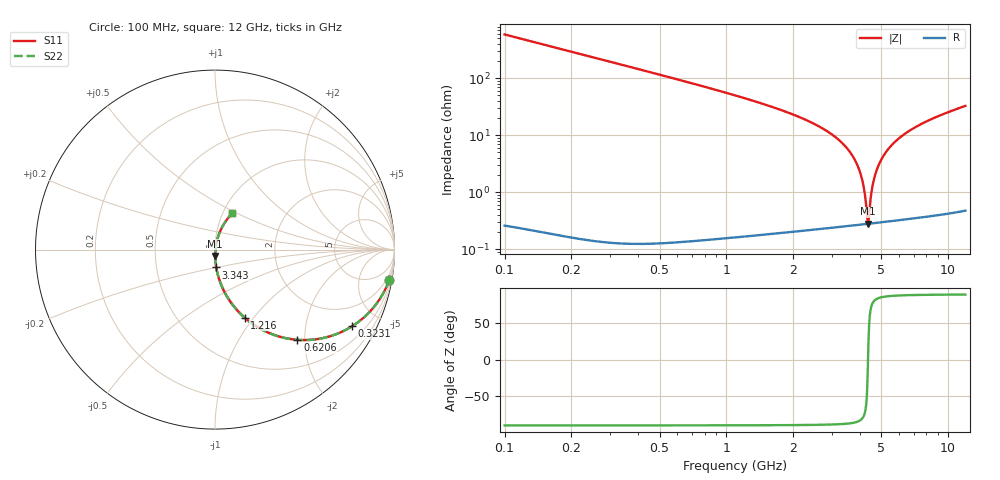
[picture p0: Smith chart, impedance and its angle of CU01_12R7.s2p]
! S-parameter model data by Modelithics Inc. support@modelithics.com 813-866-6335 Tampa FL USA
! S-Parameter data specifications:
! Substrate: 20-mil Rogers, substrate thickness, H=0.508mm, Dielectric constant, Er=3.75
! PCB Mounting Pad Footprint: Pad width, PadW=0.35mm , Pad length, PadL=0.30mm , Pad gap, PadG (edge-to-edge)=0.25mm , Reference planes=0.85mm apart
! Created Tue May  8 14:01:25 2018
# hz S ma R 50
! 2 Port Network Data from SP1.SP block
! freq  magS11  angS11  magS21  angS21  magS12  angS12  magS22  angS22
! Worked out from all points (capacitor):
!   801 points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, 100 MHz to 12 GHz, reference 50 ohm
!   read as one part in series: C = 2.72 pF near 159.5 MHz
!   lowest |Z| = 283 mohm at 4.369 GHz (marker M1)
!   series resonance near 4.363 GHz, so ESL is about 490 pH
!   S11 on the Smith chart (normalised r, x): 100 MHz: 1, -12; 323.1 MHz: 0.98, -3.58; 620.6 MHz: 0.98, -1.84; 1.216 GHz: 0.99, -0.90; 3.343 GHz: 0.99, -0.20; 12 GHz: 1.11, +0.47
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1e8  0.9857 -9.8  0.1682 80.2  0.1682 80.2  0.9857 -9.8
2.19e8  0.9364 -20.7  0.3505 69.2  0.3505 69.2  0.9364 -20.7
3.23125e8  0.8747 -29.3  0.4841 60.7  0.4841 60.7  0.8747 -29.3
6.20625e8  0.6808 -47.6  0.7315 42.3  0.7315 42.3  0.6808 -47.6
8.88375e8  0.5385 -58.1  0.8414 31.7  0.8414 31.7  0.5385 -58.1
1.215625e9  0.4136 -66.5  0.9089 23.3  0.9089 23.3  0.4136 -66.5
2.09325e9  0.2268 -78.4  0.9719 11.1  0.9719 11.1  0.2268 -78.4
3.34275e9  0.09986 -86.1  0.9925 2.5  0.9925 2.5  0.09986 -86.1
4.071625e9  0.05258 -88.0  0.9959 -0.9  0.9959 -0.9  0.05258 -88.0
4.369125e9  0.03616 -87.7  0.9965 -2.1  0.9965 -2.1  0.03616 -87.7
4.785625e9  0.01527 -82.9  0.9969 -3.7  0.9969 -3.7  0.01527 -82.9
4.9195e9  0.009111 -75.6  0.997 -4.2  0.997 -4.2  0.009111 -75.6
5.06825e9  0.003438 -35.7  0.997 -4.8  0.997 -4.8  0.003438 -35.7
5.112875e9  0.002972 0.0  0.997 -4.9  0.997 -4.9  0.002972 0.0
5.321125e9  0.00994 66.7  0.9969 -5.6  0.9969 -5.6  0.00994 66.7
5.469875e9  0.01614 73.0  0.9967 -6.1  0.9967 -6.1  0.01614 73.0
5.72275e9  0.02652 76.3  0.9965 -7.0  0.9965 -7.0  0.02652 76.3
6.05e9  0.03947 77.3  0.9959 -8.0  0.9959 -8.0  0.03947 77.3
6.85325e9  0.0691 76.7  0.9941 -10.5  0.9941 -10.5  0.0691 76.7
8.04325e9  0.1089 74.1  0.9903 -13.9  0.9903 -13.9  0.1089 74.1
1.002162e10  0.1685 69.3  0.9815 -19.3  0.9815 -19.3  0.1685 69.3
1.2e10  0.2235 64.4  0.9699 -24.4  0.9699 -24.4  0.2235 64.4
